(* Logix 5000 AddOnInstructionDefinition export YAI_Assy_155_120_EIP_Hz; software revision 21.03 *)

ADD_ON_INSTRUCTION YAI_Assy_155_120_EIP_Hz   (* revision 1.0, vendor Yaskawa America, Inc. *)
// YAI Assembly 155 and 120
// Help:
// This add-on instruction is for use with input assemblie 166 and output assemblies 116.
// Node_Input_Assy is defined as the node's input assembly integer array.
// Node_Output_Assy is defined as the node's output assembly integer array.
// Torque limit/reference, torque compensation and torque output variables are only available with A1000.
VAR_IN_OUT
   Node_Input_Assy : AB:ETHERNET_MODULE_INT_40Bytes:I:0; {required}   // Input assembly words
   Node_Output_Assy : AB:ETHERNET_MODULE_INT_24Bytes:O:0; {required}   // Output assembly words
END_VAR
VAR_INPUT
   RunFwd : BOOL; {visible}   // Forward run command
   RunRev : BOOL; {visible}   // Reverse run command
   MFI_3 : BOOL; {visible}   // Multi-function input 3
   MFI_4 : BOOL; {visible}   // Multi-function input 4
   MFI_5 : BOOL; {visible}   // Multi-function input 5
   MFI_6 : BOOL; {visible}   // Multi-function input 6
   MFI_7 : BOOL; {visible}   // Multi-function input 7
   MFI_8 : BOOL; {visible}   // Multi-function input 8
   External_Fault : BOOL;   // External fault command (EF0)
   FaultReset : BOOL; {visible}   // Fault reset command
   MFO_1 : BOOL; {visible}   // Multi-function output (M1-M2 for A/P1000, MA/MB/MC for V1000)
   MFO_2 : BOOL; {visible}   // Multi-function output (M3-M4 for A/P1000, P1 for V1000)
   MFO_3 : BOOL; {visible}   // Multi-function output (M5-M6 for A/P1000, P2 for V1000)
   Freq_Ref : REAL; {visible}   // Frequency reference command in Hz (xx.xx resolution)
   Digital_Output_Fault_Enable : BOOL;   // Bit to enable control of fault output relay over the network
END_VAR
VAR_OUTPUT
   Running : BOOL; {access Read Only, visible}   // Drive running forward status bit
   ZSP : BOOL; {access Read Only, visible}   // Drive zero speed status bit
   RunningRev : BOOL; {access Read Only, visible}   // Drive running reverse status bit
   Reset : BOOL; {access Read Only, visible}   // Drive reset command status bit
   At_Speed : BOOL; {access Read Only, visible}   // Drive at commanded speed status bit
   Ready : BOOL; {access Read Only, visible}   // Drive ready status bit
   Alarm : BOOL; {access Read Only, visible}   // Drive alarm status bit
   Faulted : BOOL; {access Read Only, visible}   // Drive faulted status bit
   OPE : BOOL; {access Read Only}   // OPE alarm/fault present
   UV : BOOL; {access Read Only}   // Drive in UV (undervoltage) state status bit
   NetCtrlStatus : BOOL; {access Read Only, visible}   // Drive network run source status bit (1 = source coming from network)
   MFO_1_Status : BOOL; {access Read Only, visible}   // Drive multi-function output 1 (M1-M2 for A/P1000, MA/MB/MC for V1000) status
   MFO_2_Status : BOOL; {access Read Only, visible}   // Drive multi-function output 1 (M3-M4 for A/P1000, P1 for V1000) status
   MFO_3_Status : BOOL; {access Read Only, visible}   // Drive multi-function output 1 (M5-M6 for A/P1000, P2 for V1000) status
   ZSV : BOOL; {access Read Only, visible}   // Drive zero servo completed status bit
   Motor_Speed : REAL; {access Read Only, visible}   // Motor speed in Hz (xx.xx resolution)
   Torque_Actual : REAL; {access Read Only, visible}   // Drive torque output in % (xxx.x resolution)
   PG1_Count : INT; {access Read Only}   // Encoder feedback count
   Freq_Cmd : REAL; {access Read Only, visible}   // Commanded frequency in Hz (xx.xx resolution)
   Output_Freq : REAL; {access Read Only, visible}   // Drive output frequency in Hz (xx.xx resolution)
   Output_Current : REAL; {access Read Only, visible}   // Drive output current in A (xxx.x resolution)
   Analog_Input_1_Level : REAL; {access Read Only}   // Analog input 1 level in % (xxx.x resolution)
   DC_Bus_Volt : INT; {access Read Only, visible}   // DC bus voltage in Vdc (xxx resolution)
   Analog_Input_3_Level : REAL; {access Read Only}   // Analog input 3 level in % (xxx.x resolution)
   Analog_Input_2_Level : REAL; {access Read Only}   // Analog input 2 level in % (xxx.x resolution)
   S1_Status : BOOL; {access Read Only}   // Digital input S1 status
   S2_Status : BOOL; {access Read Only}   // Digital input S2 status
   S3_Status : BOOL; {access Read Only}   // Digital input S3 status
   S4_Status : BOOL; {access Read Only}   // Digital input S4 status
   S5_Status : BOOL; {access Read Only}   // Digital input S5 status
   S6_Status : BOOL; {access Read Only}   // Digital input S6 status
   S7_Status : BOOL; {access Read Only}   // Digital input S7 status
   S8_Status : BOOL; {access Read Only}   // Digital input S8 status
   PG2_Count : INT;   // Encoder 2 feedback count
   UV_Alarm : BOOL; {access Read Only}   // Undervoltage alarm
   OV_Alarm : BOOL; {access Read Only}   // Overvoltage alarm
   OH_Alarm : BOOL; {access Read Only}   // Overheat alarm
   OH2_Alarm : BOOL; {access Read Only}   // Drive overheat alarm
   OL3_Alarm : BOOL; {access Read Only}   // Overtorque detection 1 alarm
   OL4_Alarm : BOOL; {access Read Only}   // Overtorque detection 2 alarm
   EF_Alarm : BOOL; {access Read Only}   // Run command error alarm
   bb_Alarm : BOOL; {access Read Only}   // Baseblock alarm
   EF3_Alarm : BOOL; {access Read Only}   // External fault 3 alarm
   EF4_Alarm : BOOL; {access Read Only}   // External fault 4 alarm
   EF5_Alarm : BOOL; {access Read Only}   // External fault 5 alarm
   EF6_Alarm : BOOL; {access Read Only}   // External fault 6 alarm
   EF7_Alarm : BOOL; {access Read Only}   // External fault 7 alarm
   EF8_Alarm : BOOL; {access Read Only}   // External fault 8 alarm
   FAN_Alarm : BOOL; {access Read Only}   // Cooling fan error alarm
   OS_Alarm : BOOL; {access Read Only}   // Overspeed alarm
   DEV_Alarm : BOOL; {access Read Only}   // Speed deviation alarm
   PGO_Alarm : BOOL; {access Read Only}   // Encoder feedback open alarm
   OPR_Alarm : BOOL; {access Read Only}   // Operator removed alarm
   CE_Alarm : BOOL; {access Read Only}   // Serial communication error alarm
   BUS_Alarm : BOOL; {access Read Only}   // BUS alarm
   CALL_Alarm : BOOL; {access Read Only}   // Serial communication timeout alarm
   OL1_Alarm : BOOL; {access Read Only}   // Motor overload alarm
   OL2_Alarm : BOOL; {access Read Only}   // Drive overload alarm
   EF0_Alarm : BOOL; {access Read Only}   // External fault 0 alarm
   RUN_Alarm : BOOL; {access Read Only}   // Motor 2 run command issued while running alarm
   UL3_Alarm : BOOL; {access Read Only}   // Undertorque detecxtion 1 alarm
   UL4_Alarm : BOOL; {access Read Only}   // Undertorque detection 2 alarm
   SE_Alarm : BOOL; {access Read Only}   // Modbus test failure alarm
   OH3_Alarm : BOOL; {access Read Only}   // Motor overload alarm
   FBL_Alarm : BOOL; {access Read Only}   // PID feedback loss alarm
   FBH_Alarm : BOOL; {access Read Only}   // PID feedback loss alarm
   DNE_Alarm : BOOL; {access Read Only}   // Drive not enabled alarm
END_VAR
VAR_INPUT
   Custom_Out_1 : INT;
   Custom_Out_2 : INT;
   Custom_Out_3 : INT;
   Custom_Out_4 : INT;
   Custom_Out_5 : INT;
   Custom_Out_6 : INT;
   Custom_Out_7 : INT;
   Custom_Out_8 : INT;
   Custom_Out_9 : INT;
   Custom_Out_10 : INT;
END_VAR
VAR
   FRef_Convert : DINT;
   FOut_Convert : REAL;
   FOut_Temp : REAL;
   TRef_Convert : INT;
   TComp_Convert : INT;
   TOut_Convert : REAL;
   TOut_Temp : REAL;
   IOut_Temp : REAL;
   IOut_Convert : REAL;
   AO1_Convert : INT;
   AO2_Convert : INT;
   Motor_Speed_Temp : REAL;
   Motor_Speed_Convert : REAL;
   Freq_Cmd_Temp : REAL;
   Freq_Cmd_Convert : REAL;
   AI1_Temp : REAL;
   AI1_Convert : REAL;
   AI2_Temp : REAL; {access None}
   AI2_Convert : REAL; {access None}
   AI3_Temp : REAL; {access None}
   AI3_Convert : REAL; {access None}
END_VAR

ROUTINE Logic   (* ladder *)
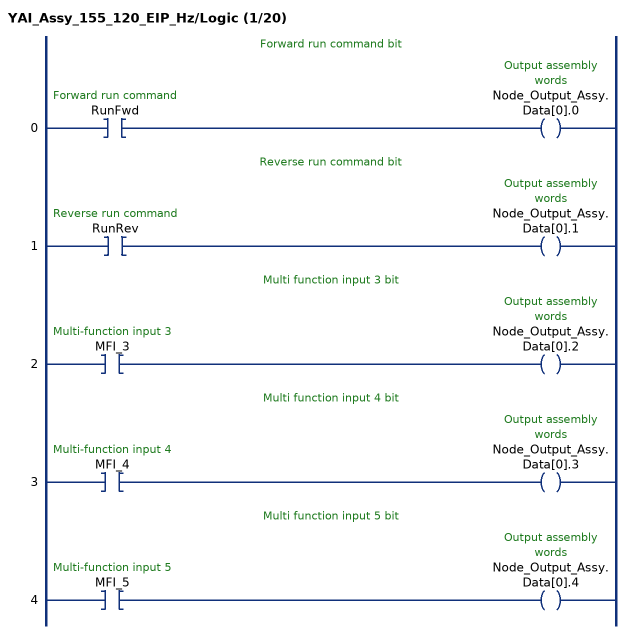
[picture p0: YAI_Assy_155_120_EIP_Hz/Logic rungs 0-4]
   // Forward run command bit
   0: XIC(RunFwd)OTE(Node_Output_Assy.Data[0].0);
   // Reverse run command bit
   1: XIC(RunRev)OTE(Node_Output_Assy.Data[0].1);
   // Multi function input 3 bit
   2: XIC(MFI_3)OTE(Node_Output_Assy.Data[0].2);
   // Multi function input 4 bit
   3: XIC(MFI_4)OTE(Node_Output_Assy.Data[0].3);
   // Multi function input 5 bit
   4: XIC(MFI_5)OTE(Node_Output_Assy.Data[0].4);
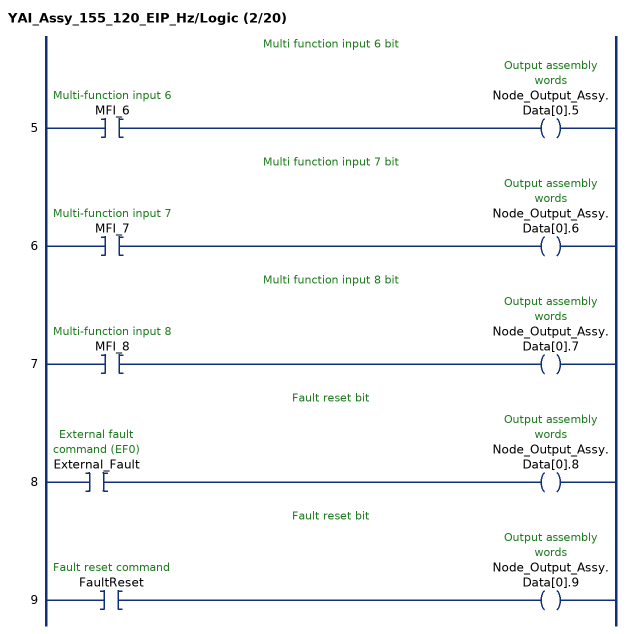
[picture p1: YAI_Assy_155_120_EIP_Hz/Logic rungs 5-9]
   // Multi function input 6 bit
   5: XIC(MFI_6)OTE(Node_Output_Assy.Data[0].5);
   // Multi function input 7 bit
   6: XIC(MFI_7)OTE(Node_Output_Assy.Data[0].6);
   // Multi function input 8 bit
   7: XIC(MFI_8)OTE(Node_Output_Assy.Data[0].7);
   // Fault reset bit
   8: XIC(External_Fault)OTE(Node_Output_Assy.Data[0].8);
   // Fault reset bit
   9: XIC(FaultReset)OTE(Node_Output_Assy.Data[0].9);
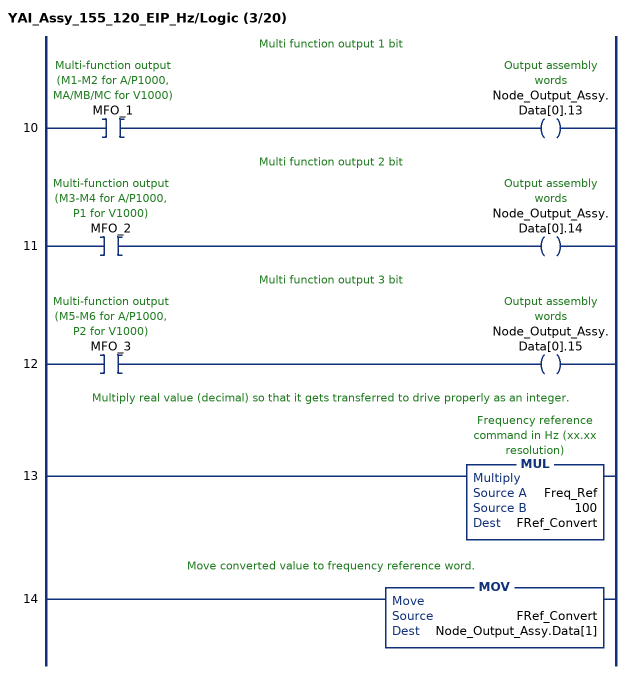
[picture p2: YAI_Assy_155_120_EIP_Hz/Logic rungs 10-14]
   // Multi function output 1 bit
   10: XIC(MFO_1)OTE(Node_Output_Assy.Data[0].13);
   // Multi function output 2 bit
   11: XIC(MFO_2)OTE(Node_Output_Assy.Data[0].14);
   // Multi function output 3 bit
   12: XIC(MFO_3)OTE(Node_Output_Assy.Data[0].15);
   // Multiply real value (decimal) so that it gets transferred to drive properly as an integer.
   13: MUL(Freq_Ref,100,FRef_Convert);
   // Move converted value to frequency reference word.
   14: MOV(FRef_Convert,Node_Output_Assy.Data[1]);
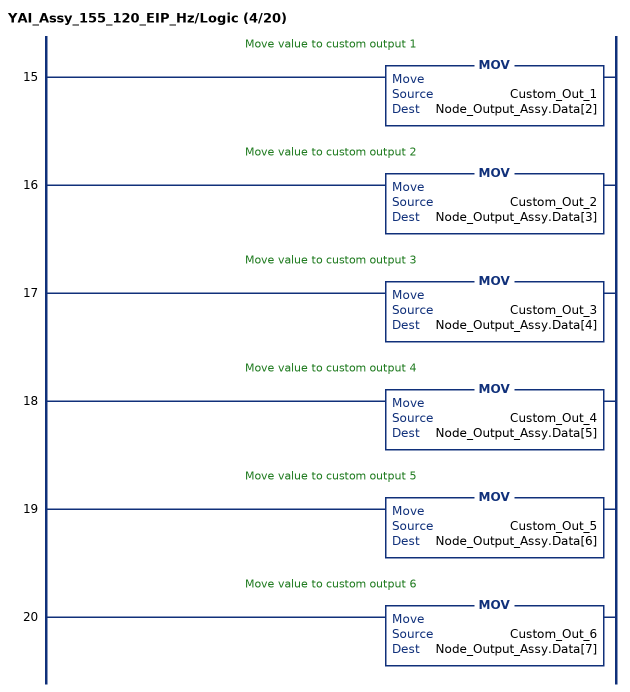
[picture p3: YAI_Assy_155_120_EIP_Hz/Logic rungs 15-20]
   // Move value to custom output 1
   15: MOV(Custom_Out_1,Node_Output_Assy.Data[2]);
   // Move value to custom output 2
   16: MOV(Custom_Out_2,Node_Output_Assy.Data[3]);
   // Move value to custom output 3
   17: MOV(Custom_Out_3,Node_Output_Assy.Data[4]);
   // Move value to custom output 4
   18: MOV(Custom_Out_4,Node_Output_Assy.Data[5]);
   // Move value to custom output 5
   19: MOV(Custom_Out_5,Node_Output_Assy.Data[6]);
   // Move value to custom output 6
   20: MOV(Custom_Out_6,Node_Output_Assy.Data[7]);
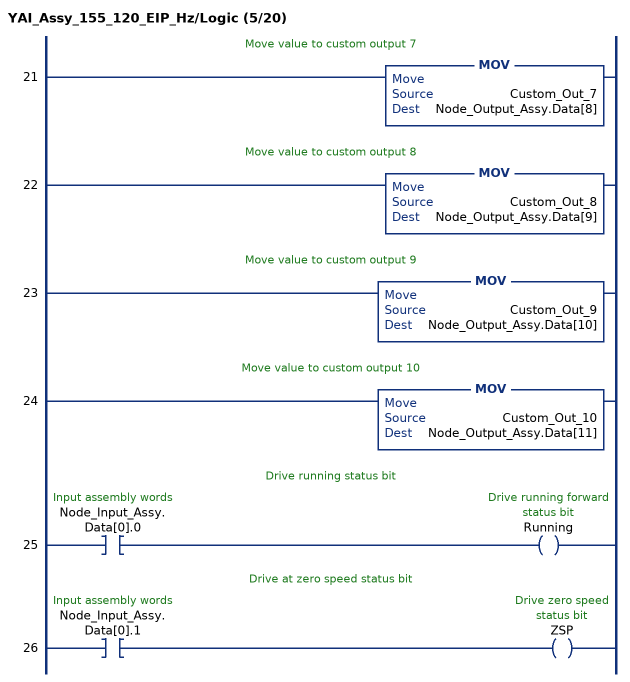
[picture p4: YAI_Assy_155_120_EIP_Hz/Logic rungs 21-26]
   // Move value to custom output 7
   21: MOV(Custom_Out_7,Node_Output_Assy.Data[8]);
   // Move value to custom output 8
   22: MOV(Custom_Out_8,Node_Output_Assy.Data[9]);
   // Move value to custom output 9
   23: MOV(Custom_Out_9,Node_Output_Assy.Data[10]);
   // Move value to custom output 10
   24: MOV(Custom_Out_10,Node_Output_Assy.Data[11]);
   // Drive running status bit
   25: XIC(Node_Input_Assy.Data[0].0)OTE(Running);
   // Drive at zero speed status bit
   26: XIC(Node_Input_Assy.Data[0].1)OTE(ZSP);
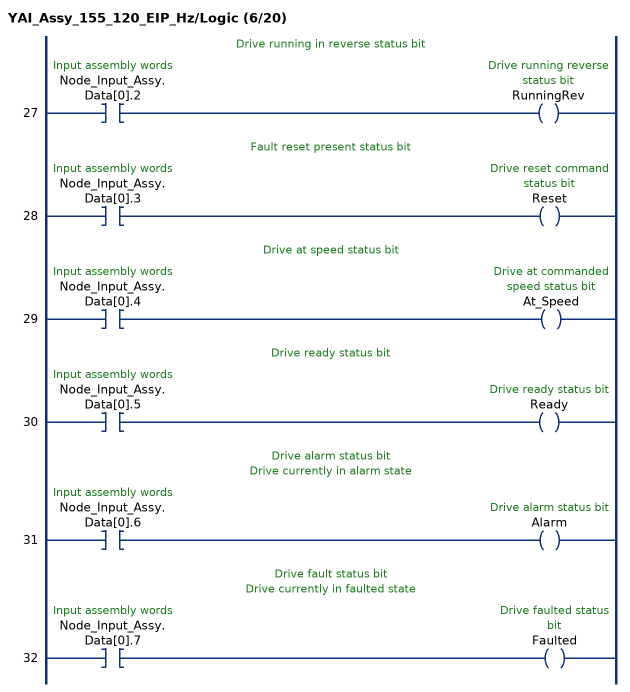
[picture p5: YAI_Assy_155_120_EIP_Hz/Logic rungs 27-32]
   // Drive running in reverse status bit
   27: XIC(Node_Input_Assy.Data[0].2)OTE(RunningRev);
   // Fault reset present status bit
   28: XIC(Node_Input_Assy.Data[0].3)OTE(Reset);
   // Drive at speed status bit
   29: XIC(Node_Input_Assy.Data[0].4)OTE(At_Speed);
   // Drive ready status bit
   30: XIC(Node_Input_Assy.Data[0].5)OTE(Ready);
   // Drive alarm status bit
   // Drive currently in alarm state
   31: XIC(Node_Input_Assy.Data[0].6)OTE(Alarm);
   // Drive fault status bit
   // Drive currently in faulted state
   32: XIC(Node_Input_Assy.Data[0].7)OTE(Faulted);
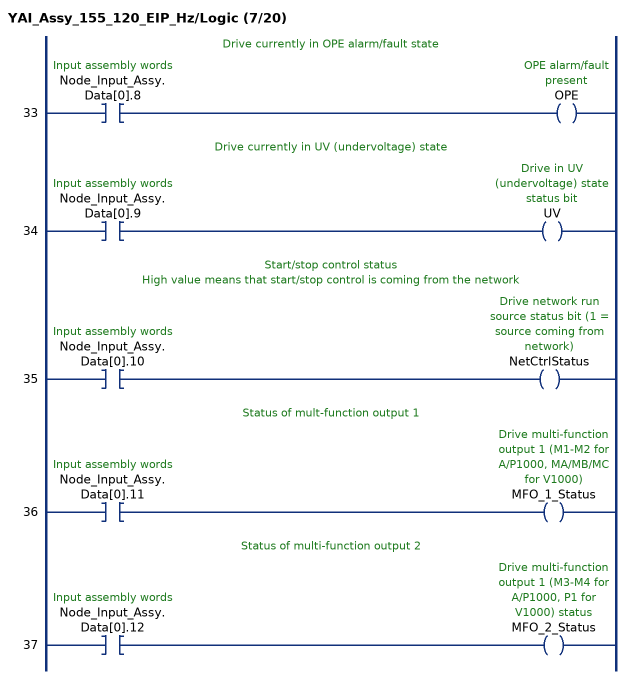
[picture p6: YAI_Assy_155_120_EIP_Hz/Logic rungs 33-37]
   // Drive currently in OPE alarm/fault state
   33: XIC(Node_Input_Assy.Data[0].8)OTE(OPE);
   // Drive currently in UV (undervoltage) state
   34: XIC(Node_Input_Assy.Data[0].9)OTE(UV);
   // Start/stop control status
   // High value means that start/stop control is coming from the network
   35: XIC(Node_Input_Assy.Data[0].10)OTE(NetCtrlStatus);
   // Status of mult-function output 1
   36: XIC(Node_Input_Assy.Data[0].11)OTE(MFO_1_Status);
   // Status of multi-function output 2
   37: XIC(Node_Input_Assy.Data[0].12)OTE(MFO_2_Status);
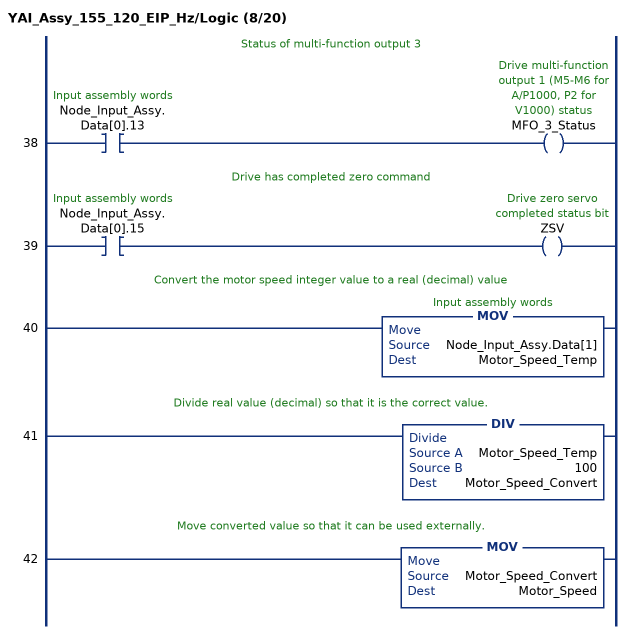
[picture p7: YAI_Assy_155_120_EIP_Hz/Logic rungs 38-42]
   // Status of multi-function output 3
   38: XIC(Node_Input_Assy.Data[0].13)OTE(MFO_3_Status);
   // Drive has completed zero command
   39: XIC(Node_Input_Assy.Data[0].15)OTE(ZSV);
   // Convert the motor speed integer value to a real (decimal) value
   40: MOV(Node_Input_Assy.Data[1],Motor_Speed_Temp);
   // Divide real value (decimal) so that it is the correct value.
   41: DIV(Motor_Speed_Temp,100,Motor_Speed_Convert);
   // Move converted value so that it can be used externally.
   42: MOV(Motor_Speed_Convert,Motor_Speed);
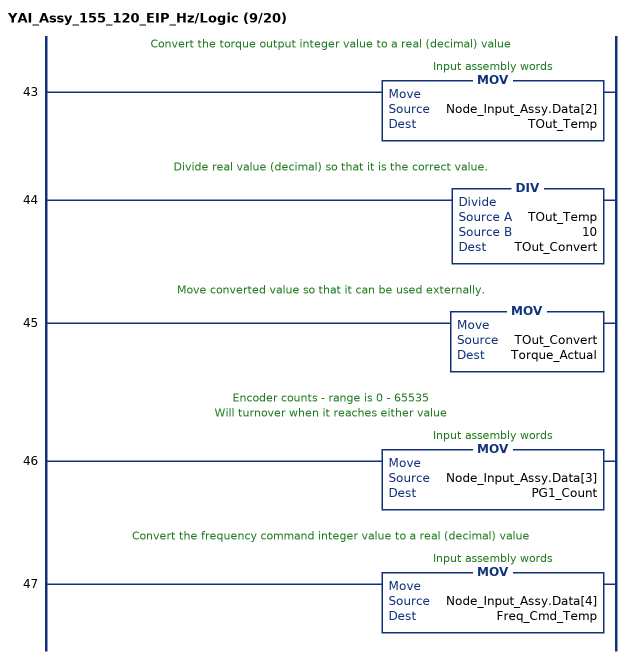
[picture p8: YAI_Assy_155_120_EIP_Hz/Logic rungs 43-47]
   // Convert the torque output integer value to a real (decimal) value
   43: MOV(Node_Input_Assy.Data[2],TOut_Temp);
   // Divide real value (decimal) so that it is the correct value.
   44: DIV(TOut_Temp,10,TOut_Convert);
   // Move converted value so that it can be used externally.
   45: MOV(TOut_Convert,Torque_Actual);
   // Encoder counts - range is 0 - 65535
   // Will turnover when it reaches either value
   46: MOV(Node_Input_Assy.Data[3],PG1_Count);
   // Convert the frequency command integer value to a real (decimal) value
   47: MOV(Node_Input_Assy.Data[4],Freq_Cmd_Temp);
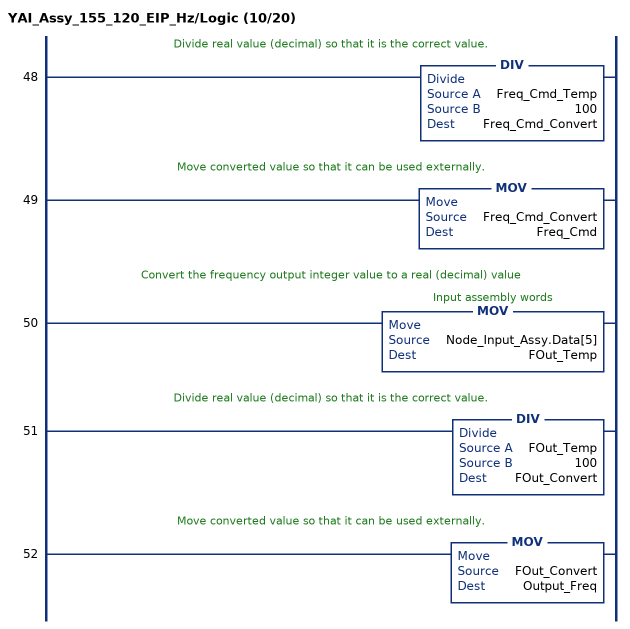
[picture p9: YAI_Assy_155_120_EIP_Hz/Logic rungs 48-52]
   // Divide real value (decimal) so that it is the correct value.
   48: DIV(Freq_Cmd_Temp,100,Freq_Cmd_Convert);
   // Move converted value so that it can be used externally.
   49: MOV(Freq_Cmd_Convert,Freq_Cmd);
   // Convert the frequency output integer value to a real (decimal) value
   50: MOV(Node_Input_Assy.Data[5],FOut_Temp);
   // Divide real value (decimal) so that it is the correct value.
   51: DIV(FOut_Temp,100,FOut_Convert);
   // Move converted value so that it can be used externally.
   52: MOV(FOut_Convert,Output_Freq);
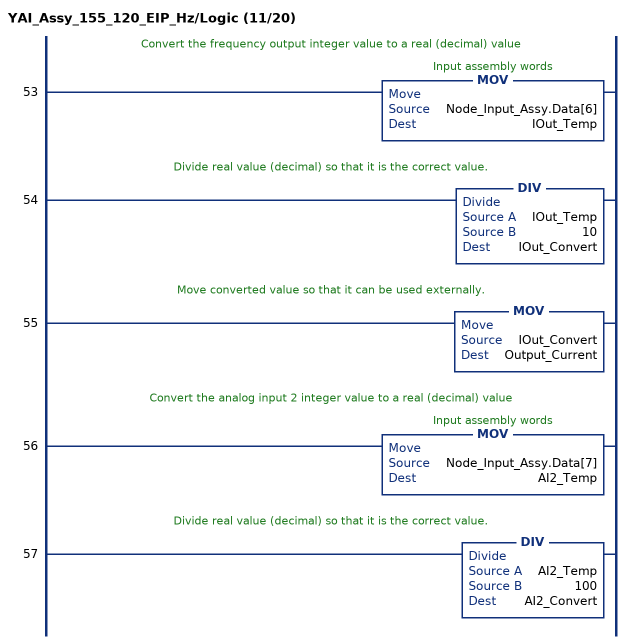
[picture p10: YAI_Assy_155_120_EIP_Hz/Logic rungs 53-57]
   // Convert the frequency output integer value to a real (decimal) value
   53: MOV(Node_Input_Assy.Data[6],IOut_Temp);
   // Divide real value (decimal) so that it is the correct value.
   54: DIV(IOut_Temp,10,IOut_Convert);
   // Move converted value so that it can be used externally.
   55: MOV(IOut_Convert,Output_Current);
   // Convert the analog input 2 integer value to a real (decimal) value
   56: MOV(Node_Input_Assy.Data[7],AI2_Temp);
   // Divide real value (decimal) so that it is the correct value.
   57: DIV(AI2_Temp,100,AI2_Convert);
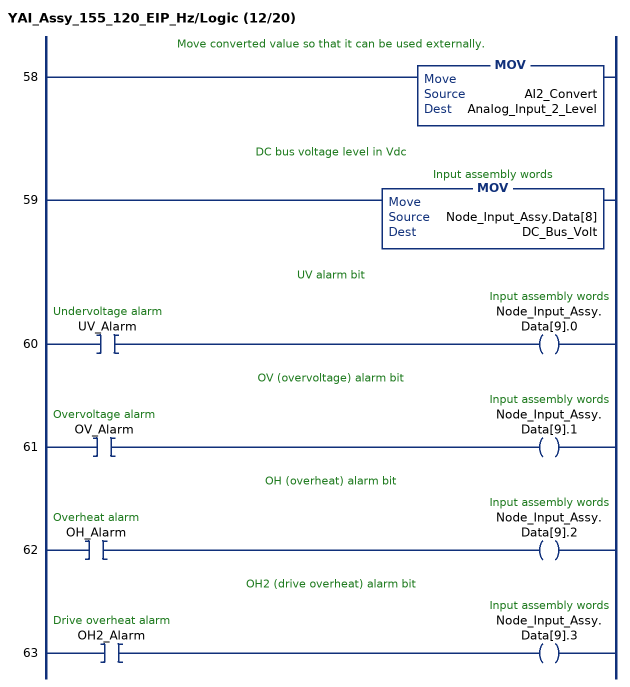
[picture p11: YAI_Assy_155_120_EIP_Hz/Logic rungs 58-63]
   // Move converted value so that it can be used externally.
   58: MOV(AI2_Convert,Analog_Input_2_Level);
   // DC bus voltage level in Vdc
   59: MOV(Node_Input_Assy.Data[8],DC_Bus_Volt);
   // UV alarm bit
   60: XIC(UV_Alarm)OTE(Node_Input_Assy.Data[9].0);
   // OV (overvoltage) alarm bit
   61: XIC(OV_Alarm)OTE(Node_Input_Assy.Data[9].1);
   // OH (overheat) alarm bit
   62: XIC(OH_Alarm)OTE(Node_Input_Assy.Data[9].2);
   // OH2 (drive overheat) alarm bit
   63: XIC(OH2_Alarm)OTE(Node_Input_Assy.Data[9].3);
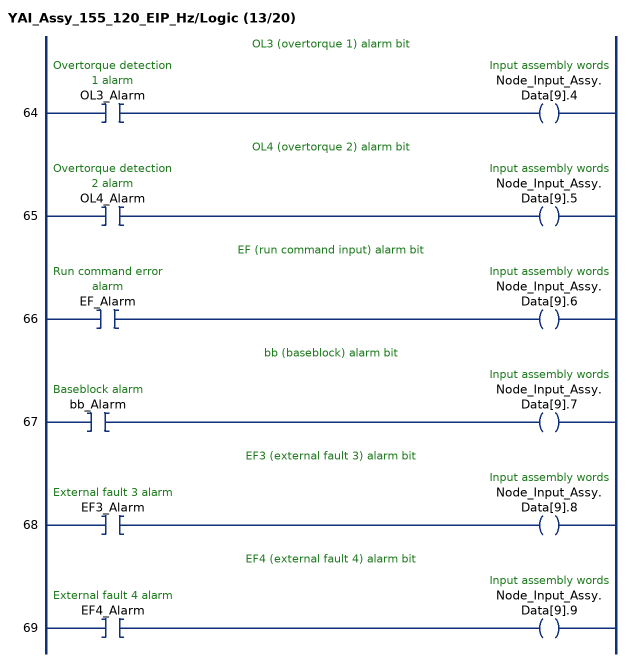
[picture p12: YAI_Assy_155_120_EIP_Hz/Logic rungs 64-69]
   // OL3 (overtorque 1) alarm bit
   64: XIC(OL3_Alarm)OTE(Node_Input_Assy.Data[9].4);
   // OL4 (overtorque 2) alarm bit
   65: XIC(OL4_Alarm)OTE(Node_Input_Assy.Data[9].5);
   // EF (run command input) alarm bit
   66: XIC(EF_Alarm)OTE(Node_Input_Assy.Data[9].6);
   // bb (baseblock) alarm bit
   67: XIC(bb_Alarm)OTE(Node_Input_Assy.Data[9].7);
   // EF3 (external fault 3) alarm bit
   68: XIC(EF3_Alarm)OTE(Node_Input_Assy.Data[9].8);
   // EF4 (external fault 4) alarm bit
   69: XIC(EF4_Alarm)OTE(Node_Input_Assy.Data[9].9);
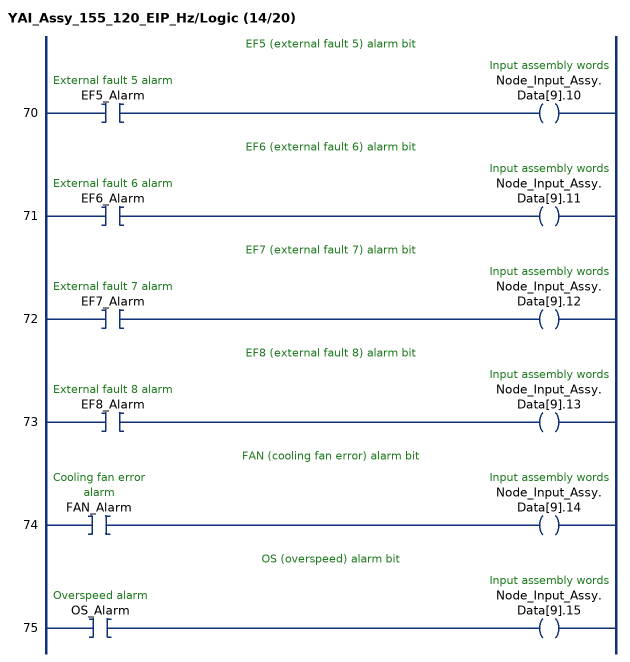
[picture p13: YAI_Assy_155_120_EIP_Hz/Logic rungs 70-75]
   // EF5 (external fault 5) alarm bit
   70: XIC(EF5_Alarm)OTE(Node_Input_Assy.Data[9].10);
   // EF6 (external fault 6) alarm bit
   71: XIC(EF6_Alarm)OTE(Node_Input_Assy.Data[9].11);
   // EF7 (external fault 7) alarm bit
   72: XIC(EF7_Alarm)OTE(Node_Input_Assy.Data[9].12);
   // EF8 (external fault 8) alarm bit
   73: XIC(EF8_Alarm)OTE(Node_Input_Assy.Data[9].13);
   // FAN (cooling fan error) alarm bit
   74: XIC(FAN_Alarm)OTE(Node_Input_Assy.Data[9].14);
   // OS (overspeed) alarm bit
   75: XIC(OS_Alarm)OTE(Node_Input_Assy.Data[9].15);
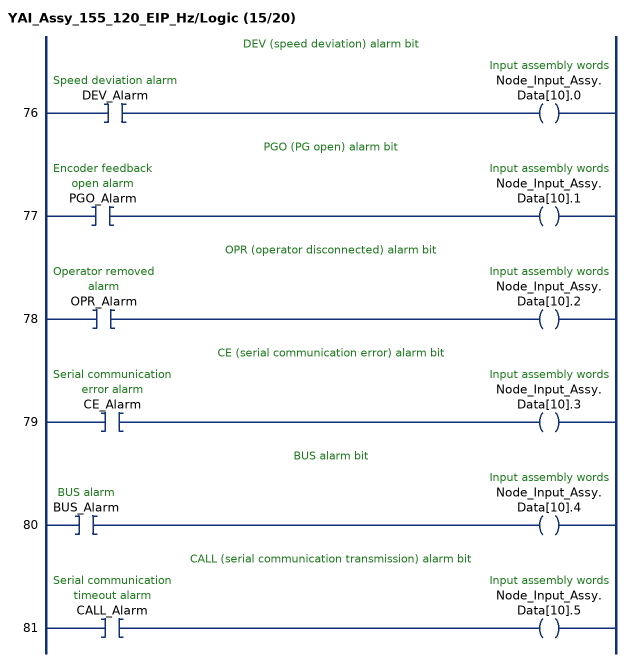
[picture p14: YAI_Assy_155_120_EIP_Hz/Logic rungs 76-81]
   // DEV (speed deviation) alarm bit
   76: XIC(DEV_Alarm)OTE(Node_Input_Assy.Data[10].0);
   // PGO (PG open) alarm bit
   77: XIC(PGO_Alarm)OTE(Node_Input_Assy.Data[10].1);
   // OPR (operator disconnected) alarm bit
   78: XIC(OPR_Alarm)OTE(Node_Input_Assy.Data[10].2);
   // CE (serial communication error) alarm bit
   79: XIC(CE_Alarm)OTE(Node_Input_Assy.Data[10].3);
   // BUS alarm bit
   80: XIC(BUS_Alarm)OTE(Node_Input_Assy.Data[10].4);
   // CALL (serial communication transmission) alarm bit
   81: XIC(CALL_Alarm)OTE(Node_Input_Assy.Data[10].5);
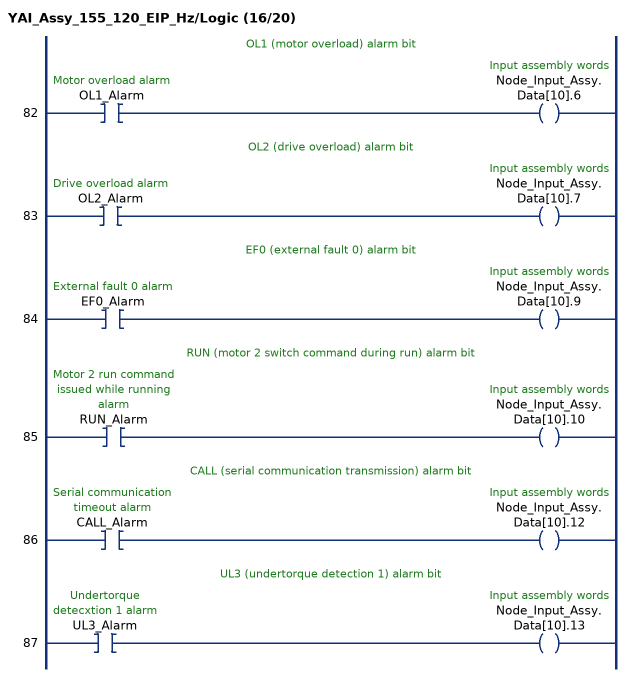
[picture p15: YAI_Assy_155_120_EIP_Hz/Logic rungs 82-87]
   // OL1 (motor overload) alarm bit
   82: XIC(OL1_Alarm)OTE(Node_Input_Assy.Data[10].6);
   // OL2 (drive overload) alarm bit
   83: XIC(OL2_Alarm)OTE(Node_Input_Assy.Data[10].7);
   // EF0 (external fault 0) alarm bit
   84: XIC(EF0_Alarm)OTE(Node_Input_Assy.Data[10].9);
   // RUN (motor 2 switch command during run) alarm bit
   85: XIC(RUN_Alarm)OTE(Node_Input_Assy.Data[10].10);
   // CALL (serial communication transmission) alarm bit
   86: XIC(CALL_Alarm)OTE(Node_Input_Assy.Data[10].12);
   // UL3 (undertorque detection 1) alarm bit
   87: XIC(UL3_Alarm)OTE(Node_Input_Assy.Data[10].13);
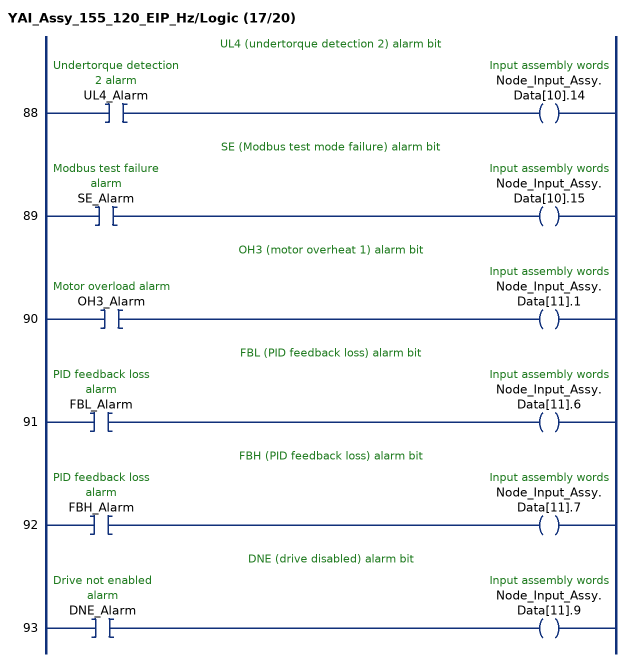
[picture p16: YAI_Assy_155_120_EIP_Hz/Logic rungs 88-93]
   // UL4 (undertorque detection 2) alarm bit
   88: XIC(UL4_Alarm)OTE(Node_Input_Assy.Data[10].14);
   // SE (Modbus test mode failure) alarm bit
   89: XIC(SE_Alarm)OTE(Node_Input_Assy.Data[10].15);
   // OH3 (motor overheat 1) alarm bit
   90: XIC(OH3_Alarm)OTE(Node_Input_Assy.Data[11].1);
   // FBL (PID feedback loss) alarm bit
   91: XIC(FBL_Alarm)OTE(Node_Input_Assy.Data[11].6);
   // FBH (PID feedback loss) alarm bit
   92: XIC(FBH_Alarm)OTE(Node_Input_Assy.Data[11].7);
   // DNE (drive disabled) alarm bit
   93: XIC(DNE_Alarm)OTE(Node_Input_Assy.Data[11].9);
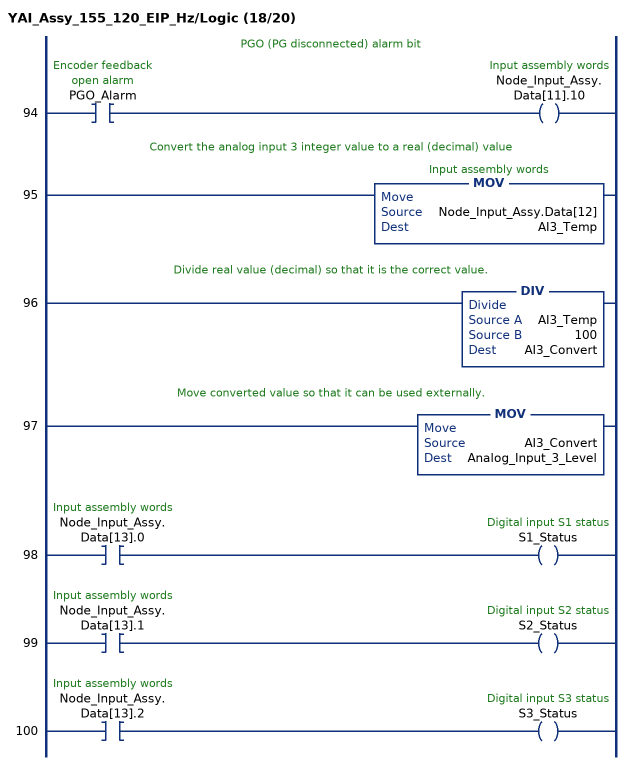
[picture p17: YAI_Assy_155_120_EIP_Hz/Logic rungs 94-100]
   // PGO (PG disconnected) alarm bit
   94: XIC(PGO_Alarm)OTE(Node_Input_Assy.Data[11].10);
   // Convert the analog input 3 integer value to a real (decimal) value
   95: MOV(Node_Input_Assy.Data[12],AI3_Temp);
   // Divide real value (decimal) so that it is the correct value.
   96: DIV(AI3_Temp,100,AI3_Convert);
   // Move converted value so that it can be used externally.
   97: MOV(AI3_Convert,Analog_Input_3_Level);
   98: XIC(Node_Input_Assy.Data[13].0)OTE(S1_Status);
   99: XIC(Node_Input_Assy.Data[13].1)OTE(S2_Status);
   100: XIC(Node_Input_Assy.Data[13].2)OTE(S3_Status);
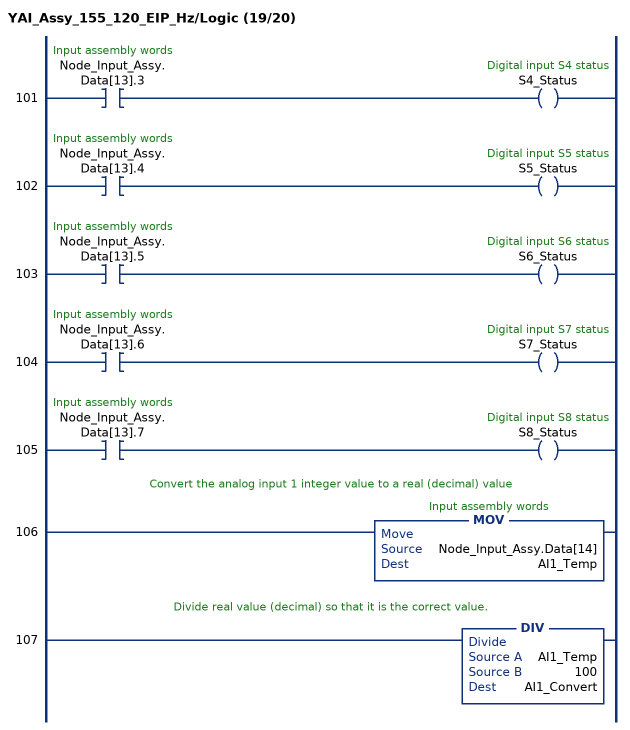
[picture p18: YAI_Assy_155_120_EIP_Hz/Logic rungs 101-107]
   101: XIC(Node_Input_Assy.Data[13].3)OTE(S4_Status);
   102: XIC(Node_Input_Assy.Data[13].4)OTE(S5_Status);
   103: XIC(Node_Input_Assy.Data[13].5)OTE(S6_Status);
   104: XIC(Node_Input_Assy.Data[13].6)OTE(S7_Status);
   105: XIC(Node_Input_Assy.Data[13].7)OTE(S8_Status);
   // Convert the analog input 1 integer value to a real (decimal) value
   106: MOV(Node_Input_Assy.Data[14],AI1_Temp);
   // Divide real value (decimal) so that it is the correct value.
   107: DIV(AI1_Temp,100,AI1_Convert);
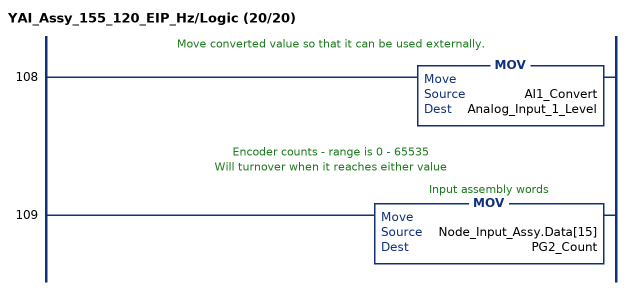
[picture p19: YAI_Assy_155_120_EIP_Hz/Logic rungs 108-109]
   // Move converted value so that it can be used externally.
   108: MOV(AI1_Convert,Analog_Input_1_Level);
   // Encoder counts - range is 0 - 65535
   // Will turnover when it reaches either value
   109: MOV(Node_Input_Assy.Data[15],PG2_Count);
END_ROUTINE
END_ADD_ON_INSTRUCTION
